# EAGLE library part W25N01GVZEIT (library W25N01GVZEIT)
1Gb QspiNAND Flash 104MHz SON8 Source: Datasheet
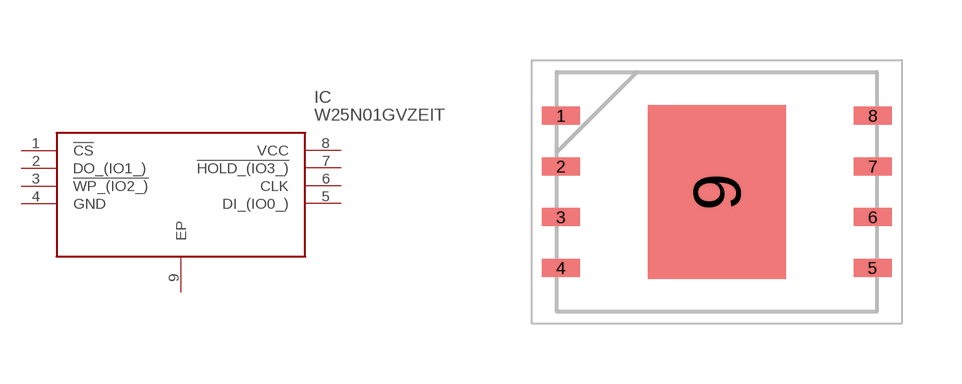
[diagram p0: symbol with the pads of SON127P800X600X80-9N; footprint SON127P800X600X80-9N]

Designator prefix IC

## W25N01GVZEIT (Arrow_Part_Number: W25N01GVZEIT; Arrow_Price-Stock: https://www.arrow.com/en/products/w25n01gvzeit/winbond-electronics?region=nac; Description: 1Gb QspiNAND Flash 104MHz SON8; Height: 0.8mm; Manufacturer_Name: Winbond; Manufacturer_Part_Number: W25N01GVZEIT; Mouser_Part_Number: 454-W25N01GVZEIT; Mouser_Price-Stock: https://www.mouser.co.uk/ProductDetail/Winbond/W25N01GVZEIT?qs=qSfuJ%252Bfl%2Fd62yqJfJtnOQw%3D%3D)  [SON127P800X600X80-9N]
1  !CS
2  DO_(IO1_)
3  !WP_(IO2_)
4  GND
5  DI_(IO0_)
6  CLK
7  !HOLD_(IO3_)
8  VCC
9  EP

## Footprint SON127P800X600X80-9N (pad centres in mm)
8-Pad WSON 8x6-mm (Package Code ZE)
smd 0.95 x 0.45: 1 -3.9,1.905; 2 -3.9,0.635; 3 -3.9,-0.635; 4 -3.9,-1.905; 5 3.9,-1.905; 6 3.9,-0.635; 7 3.9,0.635; 8 3.9,1.905
smd 3.45 x 4.35: 9 0,0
